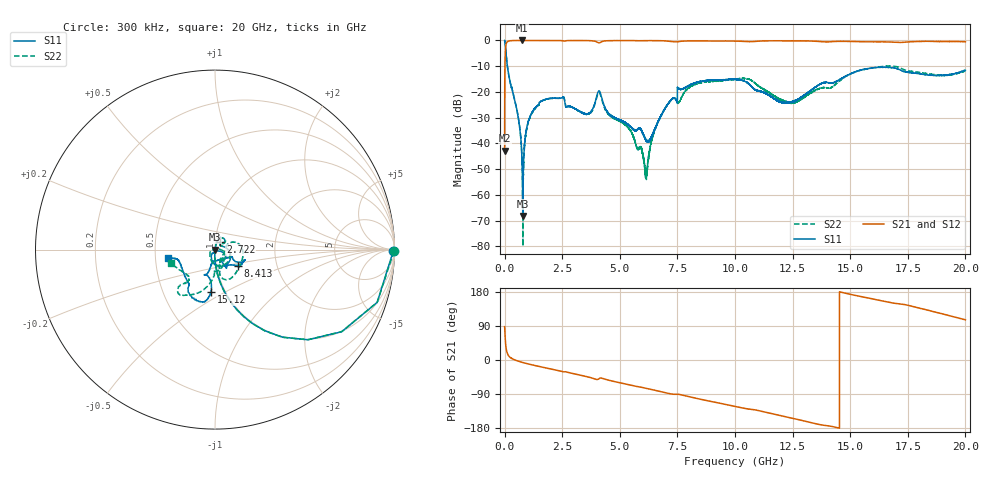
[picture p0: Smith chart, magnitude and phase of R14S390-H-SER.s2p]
!{R14S390}
!Johanson Technology Inc.
!www.johansontechnology.com
!Test Board Conditions:
!Substrate Type  RO4350B
!Substrate Thickness  20 mil
!Substrate Dk  3.66
!TL Type: GCPW
!TL Trace Width  36 mil
!TL Gap  12 mil
!Electrode orientation  Horizontal
!DUT TOPOLOGY	SERIES
!Mounting Pad LxW  26x36 mil
! Created Wed Nov 25 17:33:21 2020
! 2 Port Network Data from SP1.SP block
! freq  magS11  angS11  magS21  angS21  magS12  angS12  magS22  angS22
# khz S ma R 50
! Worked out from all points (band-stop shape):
!   20001 points, 300 kHz to 20 GHz, reference 50 ohm
!   highest |S21| = 0.00 dB at 760.3 MHz (marker M1); lowest = -42.8 dB at 300 kHz (marker M2)
!   |S21| within 3 dB of the highest: 41.21 MHz to end of sweep
!   lowest |S11| = -68.2 dB at 791.3 MHz (marker M3), VSWR 1.00, Z = 50 + j0.0104 ohm
!   |S11| at or under -10 dB: 120.4 MHz to end of sweep
!   |S22| runs from -79.9 to 0.0 dB; largest |S21 - S12| = 0.018
!   S11 on the Smith chart (normalised r, x): 300 kHz: open; 2.722 GHz: 1.06, +0.09; 8.413 GHz: 1.27, -0.23; 15.12 GHz: 0.86, -0.43; 20 GHz: 0.58, -0.06
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300  0.9927 -0.6  0.007241 88.2  0.007267 89.0  0.9969 -0.6
123300  0.3088 -72.9  0.9499 16.9  0.9492 16.9  0.3101 -72.9
589300  0.03236 -92.2  0.9979 -3.0  0.9982 -3.0  0.03315 -92.7
760300  0.004016 -90.4  0.9999 -6.2  0.9979 -6.1  0.004807 -94.6
791300  0.0003896 15.5  0.9983 -6.7  0.999 -6.7  0.0003518 -50.7
1010300  0.02496 78.3  0.998 -10.1  0.9986 -10.1  0.0242 79.4
1323300  0.04831 74.4  0.9968 -14.6  0.9964 -14.6  0.04769 74.8
2722300  0.05188 54.4  0.9921 -32.2  0.9923 -32.2  0.05194 49.3
3334300  0.04006 46.2  0.9947 -40.7  0.9956 -40.7  0.03972 44.3
4121300  0.1034 -61.9  0.9001 -48.5  0.9002 -48.5  0.09722 -63.6
4534300  0.03718 -122.4  0.9893 -53.5  0.9895 -53.5  0.03596 -142.4
5455300  0.02132 -123.5  0.9936 -66.1  0.9936 -66.1  0.01789 -175.7
6135300  0.01148 -89.6  0.9913 -74.6  0.9914 -74.6  0.002488 108.9
6667300  0.02698 -19.7  0.99 -81.9  0.9898 -81.9  0.02696 3.8
7600300  0.1138 -55.7  0.9573 -91.0  0.9572 -91.0  0.06603 16.8
8413300  0.1556 -34.7  0.9803 -102.4  0.9781 -102.4  0.1463 6.1
1.00003e7  0.176 -19.4  0.9708 -122.5  0.9707 -122.5  0.1773 -52.1
1.21193e7  0.06281 -69.3  0.9835 -149.0  0.9858 -149.0  0.06751 -60.8
1.33343e7  0.1107 -105.1  0.9728 -165.7  0.9742 -165.8  0.09777 -62.9
1.51203e7  0.2361 -95.3  0.9543 171.7  0.9583 171.5  0.2366 -106.9
1.66673e7  0.2971 -111.2  0.9368 152.6  0.9286 152.4  0.3195 -127.6
2e7  0.2658 -170.0  0.9434 105.9  0.9425 106.0  0.2573 -162.7
